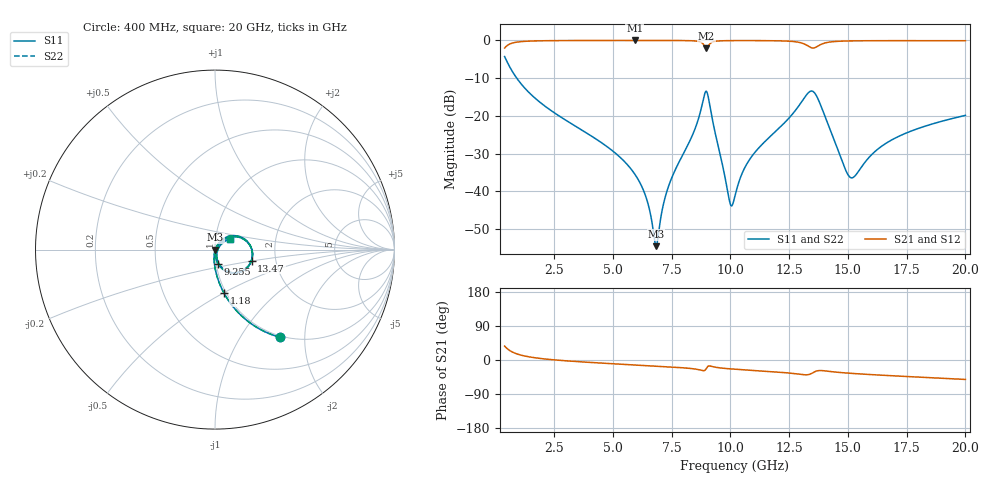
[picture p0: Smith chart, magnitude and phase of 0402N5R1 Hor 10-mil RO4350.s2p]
# GHz S MA R 50
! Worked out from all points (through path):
!   1960 points, 400 MHz to 20 GHz, reference 50 ohm
!   highest |S21| = -0.02 dB at 5.933 GHz (marker M1); lowest = -2.1 dB at 8.984 GHz (marker M2)
!   group delay of S21, straight-line fit = 8.48 ps
!   lowest |S11| = -54.6 dB at 6.843 GHz (marker M3), VSWR 1.00, Z = 50.2 - j0.0592 ohm
!   |S11| at or under -10 dB: 914.8 MHz to end of sweep
!   |S22| runs from -54.6 to -4.3 dB; largest |S21 - S12| = 0
!   S11 on the Smith chart (normalised r, x): 400 MHz: 0.98, -1.52; 1.18 GHz: 0.98, -0.51; 9.255 GHz: 1.02, -0.17; 13.47 GHz: 1.50, -0.19; 20 GHz: 1.17, +0.14
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0.4  0.6104 -53.3  0.7916 36.7  0.7916 36.7  0.6104 -53.3
0.7301685  0.3869 -68.9  0.9214 21.0  0.9214 21.0  0.3869 -68.9
1.180398  0.248 -78.3  0.9679 11.6  0.9679 11.6  0.248 -78.3
3.671669  0.06504 -94.0  0.9966 -5.0  0.9966 -5.0  0.06504 -94.0
5.932823  0.01693 -98.0  0.9981 -13.1  0.9981 -13.1  0.01693 -98.0
6.433078  0.008017 -92.8  0.998 -14.7  0.998 -14.7  0.008017 -92.8
6.843287  0.001868 -18.4  0.9978 -16.1  0.9978 -16.1  0.001868 -18.4
6.943338  0.002731 28.4  0.9978 -16.5  0.9978 -16.5  0.002731 28.4
7.373558  0.01165 60.2  0.9972 -18.0  0.9972 -18.0  0.01165 60.2
8.414089  0.05766 56.5  0.9876 -23.1  0.9876 -23.1  0.05766 56.5
8.764267  0.1254 38.1  0.9407 -27.2  0.9407 -27.2  0.1254 38.1
8.98438  0.2112 -18.4  0.7887 -21.9  0.7887 -21.9  0.2112 -18.4
9.254518  0.08429 -77.3  0.9545 -17.6  0.9545 -17.6  0.08429 -77.3
9.974885  0.007203 -42.8  0.9928 -23.3  0.9928 -23.3  0.007203 -42.8
10.205  0.008802 25.6  0.9939 -24.3  0.9939 -24.3  0.008802 25.6
10.92537  0.02928 52.8  0.9941 -27.2  0.9941 -27.2  0.02928 52.8
12.95641  0.1413 30.2  0.9377 -37.7  0.9377 -37.7  0.1413 30.2
13.46667  0.2131 -16.7  0.795 -35.2  0.795 -35.2  0.2131 -16.7
14.04696  0.09511 -72.0  0.9278 -28.9  0.9278 -28.9  0.09511 -72.0
15.1075  0.01522 -26.3  0.9843 -35.1  0.9843 -35.1  0.01522 -26.3
16.73834  0.04545 40.4  0.9916 -41.1  0.9916 -41.1  0.04545 40.4
20  0.1013 36.2  0.9897 -51.3  0.9897 -51.3  0.1013 36.2
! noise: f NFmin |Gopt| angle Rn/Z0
0.4  0.001262  0.7875  2.227  0.001222
2.571  0.004225  0.6264  6.786  0.00211
4.752  0.006558  0.5715  11.61  0.002742
6.933  0.009685  0.5774  16.35  0.004084
9.104  0.08723  0.9254  21.42  0.2502
11.29  0.02072  0.6662  26.21  0.01132
13.47  0.1472  0.9356  31.3  0.4722
15.64  0.03255  0.7057  36.06  0.0197
17.82  0.02516  0.5991  40.37  0.01027
20  0.02424  0.5533  44.45  0.00843
